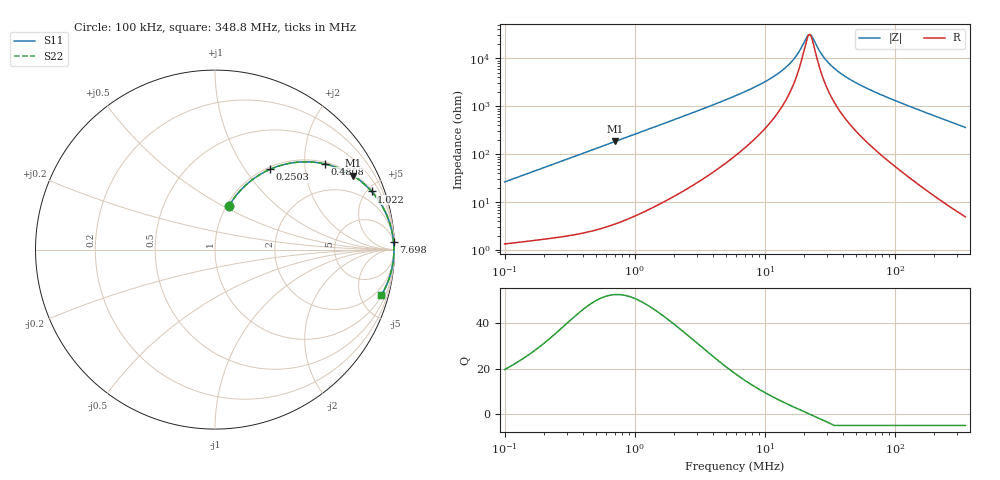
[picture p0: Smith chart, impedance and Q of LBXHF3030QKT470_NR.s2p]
! LBXHF3030QKT470_NR  S-PARAMETER MODEL  ( General Type )
! Model Generated by TAIYO YUDEN Corporation (http://www.ty-top.com)
! Version 1.0
! TAIYO YUDEN Control No. 210113NI43SB-FBB
! Copyright(c) 2021 TAIYO YUDEN CO.,LTD. All Rights Reserved.
! Product Description (link to TY-COMPAS)
! https://ds.yuden.co.jp/TYCOMPAS/or/detail?pn=LBXHF3030QKT470MNR&u=M
! Products Name : Inductors
! Characteristics :
!  Inductance : 47 uH , SRF(min) : 5.0 MHz , DC Resistance(max) : 0.98 Ohm
!  Rated Current : Saturation :290 mA , Temp Rise : 380 mA
!  Case Size : 3.0 x 3.0 / 0.118 x 0.118 [mm/inch] , Thickness : 1.5 / 0.059 [mm/inch]
!  (Conditions: Temperature = 25 degC , DC Bias Current/Voltage = 0A / 0V)
! External Node Assignments :
!  1  o---GGG---o  2
! GND o---------o GND
! Frequency Range : 0.1MHz  -  348.750116MHz  [ 402 STEP ]
# MHz S RI R 50
! Freq[MHz].  S11 Real  S11 Imag  S21 Real  S21 Imag  S12 Real  S12 Imag  S22 Real  S22 Imag
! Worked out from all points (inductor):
!   401 points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, 100 kHz to 348.8 MHz, reference 50 ohm
!   read as one part in series: L = 42.1 uH near 104.2 kHz
!   highest Q = 52.5 at 708.3 kHz (marker M1), where L = 41.6 uH
!   self-resonance near 21.78 MHz
!   S11 on the Smith chart (normalised r, x): 100 kHz: 1.03, +0.53; 250.3 kHz: 1.04, +1.32; 480.8 kHz: 1.05, +2.52; 1.022 MHz: 1.11, +5.35; 7.698 MHz: 4, +45; 348.8 MHz: 1.10, -7.27
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0.1  0.0766 0.2416  0.9234 -0.2416  0.9234 -0.2416  0.0766 0.2416
0.159843  0.1602 0.3486  0.8398 -0.3486  0.8398 -0.3486  0.1602 0.3486
0.250342  0.3071 0.4475  0.6929 -0.4475  0.6929 -0.4475  0.3071 0.4475
0.392077  0.5135 0.489  0.4865 -0.489  0.4865 -0.489  0.5135 0.489
0.480766  0.6111 0.4774  0.3889 -0.4774  0.3889 -0.4774  0.6111 0.4774
0.708278  0.7702 0.4113  0.2298 -0.4113  0.2298 -0.4113  0.7702 0.4113
1.02239  0.8725 0.3238  0.1275 -0.3238  0.1275 -0.3238  0.8725 0.3238
1.537242  0.9372 0.2317  0.0628 -0.2317  0.0628 -0.2317  0.9372 0.2317
5.905507  0.993 0.0601  0.00703 -0.0601  0.00703 -0.0601  0.993 0.0601
7.698195  0.9948 0.0437  0.00521 -0.0437  0.00521 -0.0437  0.9948 0.0437
10.88794  0.9961 0.0267  0.00393 -0.0267  0.00393 -0.0267  0.9961 0.0267
13.90661  0.9965 0.0166  0.00346 -0.0166  0.00346 -0.0166  0.9965 0.0166
17.40365  0.9968 0.00836  0.00324 -0.00836  0.00324 -0.00836  0.9968 0.00836
21.34043  0.9968 0.00119  0.00316 -0.00119  0.00316 -0.00119  0.9968 0.00119
22.22879  0.9968 -0.000229  0.00316 0.000229  0.00316 0.000229  0.9968 -0.000229
23.15412  0.9968 -0.00165  0.00316 0.00165  0.00316 0.00165  0.9968 -0.00165
28.39169  0.9968 -0.00883  0.00323 0.00883  0.00323 0.00883  0.9968 -0.00883
36.26324  0.9965 -0.018  0.00347 0.018  0.00347 0.018  0.9965 -0.018
52.34555  0.9957 -0.0338  0.0043 0.0338  0.0043 0.0338  0.9957 -0.0338
90.78195  0.9923 -0.0669  0.00769 0.0669  0.00769 0.0669  0.9923 -0.0669
181.5989  0.9772 -0.138  0.0228 0.138  0.0228 0.138  0.9772 -0.138
348.7501  0.9266 -0.254  0.0734 0.254  0.0734 0.254  0.9266 -0.254
